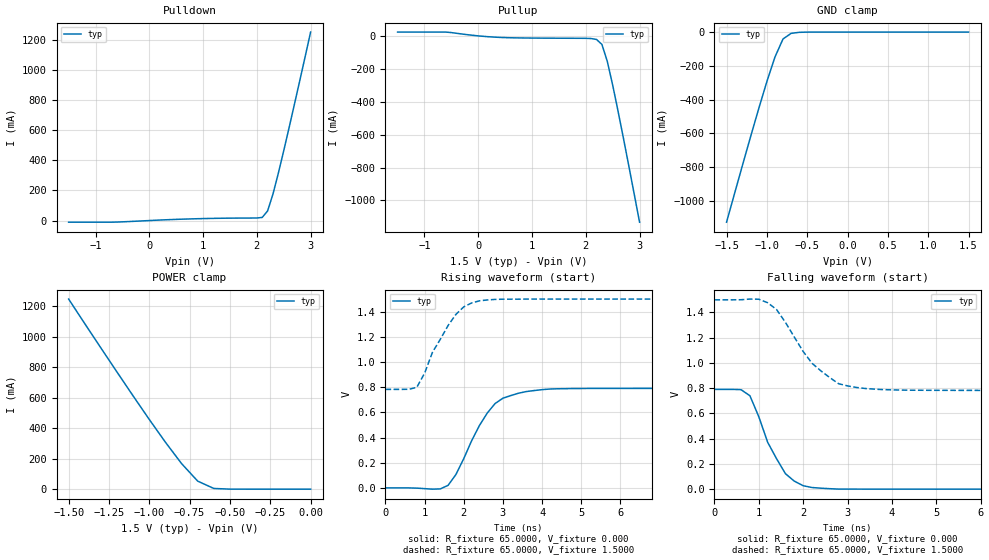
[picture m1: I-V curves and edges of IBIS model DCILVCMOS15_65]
| / 7\'7
| \ \   Xilinx Inc.
| / /
| \_\/.\   IBIS Model for Virtex-II
[IBIS ver]   2.1
[File name]   dci1565.ibs
[File Rev]   1.1
[Date]   Aug. 1, 2001
[Source]   Hspice simulations (08-01: TT, SS, FF)
[Notes]   Xilinx IBIS model for LVDCI 1.5V 65 ohms driver
[Disclaimer] The data in this model is derived from SPICE simulations using
   modeling information extracted from the target process. While
   a great deal of care has been taken to provide information
   that is accurate, this model is considered preliminary as it
   has not been verified by actual silicon measurement. Treat the
   data in this model as preliminary until actual silicon
   verification is performed.
[Copyright]   Copyright 2001, Xilinx Inc., All rights reserved
|   Component Virtex_II
[Component]   Virtex_II
[Manufacturer]   Xilinx Inc.
[Package]
| variable   typ   min   max
R_pkg   0.1000   NA   NA
L_pkg   0.8000nH   NA   NA
C_pkg   0.5000pF   NA   NA
[Pin]  signal_name   model_name   R_pin   L_pin   C_pin
io   DCILVCMOS15_65   DCILVCMOS15_65
| ins  insig   inp
| ens  ensig   inp
PGND   GND   GND
VCCO   VCCO   POWER
| Models and submodels in the file (1): DCILVCMOS15_65 (I/O)
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|   Model DCILVCMOS15_65
[Model]   DCILVCMOS15_65
Model_type   I/O
Polarity   Non-Inverting
Enable   Active-Low
Vinh = 1.05V
Vinl = 0.3V
Vmeas =   0.7300V
Cref =  35.0000pF
Rref =   1.0000M
Vref =  0.000V
C_comp   7.0000pF   NA   NA
[Temperature Range]   25.0000   NA   NA
[Voltage Range]   1.5000V   NA   NA
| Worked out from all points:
|   slope of the pulldown table from 0 to 0.225 V, typ, clamps not added: 58.8 ohm
|   slope of the pullup table from 0 to 0.225 V, typ, clamps not added: 37.5 ohm
|   GND clamp passes 1 mA (typ) near -0.57 V on its own axis
|   POWER clamp passes 1 mA (typ) near -0.52 V on its own axis
|   rising waveform, R_fixture 65.0000, V_fixture 0.000: 20-80 % time 819ps typ, NA min, NA max; typ from 0 V to 0.79 V
|   rising waveform, R_fixture 65.0000, V_fixture 1.5000: 20-80 % time 732ps typ, NA min, NA max; typ from 0.782 V to 1.5 V
|   falling waveform, R_fixture 65.0000, V_fixture 0.000: 20-80 % time 611ps typ, NA min, NA max; typ from 0.79 V to 0 V
|   falling waveform, R_fixture 65.0000, V_fixture 1.5000: 20-80 % time 911ps typ, NA min, NA max; typ from 1.5 V to 0.782 V
[Pulldown]
| voltage   I(typ)   I(min)   I(max)
-1.5V     -10.89mA   NA         NA
-700mV    -10.89mA   NA         NA
700mV     10.17mA    NA         NA
2.1V      20.64mA    NA         NA
2.2V      63.82mA    NA         NA
2.3V      175.9mA    NA         NA
2.4V      314.8mA    NA         NA
2.6V      617.3mA    NA         NA
3V        1.252A     NA         NA
[Pullup]
| voltage   I(typ)   I(min)   I(max)
-1.5V     22.99mA    NA         NA
-600mV    22.99mA    NA         NA
0V        -4.6nA     NA         NA
400mV     -9.254mA   NA         NA
2V        -14.9mA    NA         NA
2.2V      -21.92mA   NA         NA
2.3V      -52.01mA   NA         NA
2.4V      -155.2mA   NA         NA
2.5V      -299.2mA   NA         NA
2.6V      -457.5mA   NA         NA
2.8V      -790.2mA   NA         NA
3V        -1.132A    NA         NA
[GND_clamp]
| voltage   I(typ)   I(min)   I(max)
-1.5V     -1.127A    NA         NA
-1.2V     -617mA     NA         NA
-1V       -293.4mA   NA         NA
-900mV    -148mA     NA         NA
-800mV    -41mA      NA         NA
-700mV    -7.588mA   NA         NA
-600mV    -1.413mA   NA         NA
1.5V      218.4nA    NA         NA
[POWER_clamp]
| voltage   I(typ)   I(min)   I(max)
-1.5V     1.246A     NA         NA
-1.1V     610.9mA    NA         NA
-900mV    307.7mA    NA         NA
-800mV    167.8mA    NA         NA
-700mV    52.78mA    NA         NA
-600mV    4.607mA    NA         NA
0V        218.4nA    NA         NA
[Ramp]
| variable   typ   min   max
dV/dt_r   0.4743/0.8211n   NA   NA
dV/dt_f   0.4305/0.9045n   NA   NA
R_load = 65.0000
[Rising Waveform]
R_fixture = 65.0000
V_fixture = 0.000
| time   V(typ)   V(min)   V(max)
0s        10.73uV    NA         NA
1.4ns     -8.408mV   NA         NA
1.6ns     20.23mV    NA         NA
1.8ns     106.7mV    NA         NA
2.2ns     373.9mV    NA         NA
2.6ns     594.6mV    NA         NA
3ns       712.4mV    NA         NA
3.4ns     752.2mV    NA         NA
4.4ns     787.3mV    NA         NA
10ns      790.5mV    NA         NA
[Rising Waveform]
R_fixture = 65.0000
V_fixture = 1.5000
V_fixture_min = 1.4000
V_fixture_max = 1.6000
| time   V(typ)   V(min)   V(max)
0s        782.5mV    NA         NA
800ps     798.9mV    NA         NA
1ns       911.4mV    NA         NA
1.2ns     1.077V     NA         NA
1.6ns     1.29V      NA         NA
1.8ns     1.379V     NA         NA
2ns       1.438V     NA         NA
2.4ns     1.486V     NA         NA
3ns       1.499V     NA         NA
10ns      1.5V       NA         NA
[Falling Waveform]
R_fixture = 65.0000
V_fixture = 0.000
| time   V(typ)   V(min)   V(max)
0s        790.5mV    NA         NA
600ps     788.2mV    NA         NA
800ps     739.8mV    NA         NA
1ns       573.8mV    NA         NA
1.2ns     371.1mV    NA         NA
1.4ns     241.4mV    NA         NA
1.6ns     122.7mV    NA         NA
2ns       27.27mV    NA         NA
2.8ns     594.3uV    NA         NA
10ns      -6.526uV   NA         NA
[Falling Waveform]
R_fixture = 65.0000
V_fixture = 1.5000
V_fixture_min = 1.4000
V_fixture_max = 1.6000
| time   V(typ)   V(min)   V(max)
0s        1.5V       NA         NA
1ns       1.505V     NA         NA
1.2ns     1.477V     NA         NA
1.4ns     1.423V     NA         NA
2ns       1.091V     NA         NA
2.2ns     997.3mV    NA         NA
2.8ns     835.1mV    NA         NA
3ns       818.2mV    NA         NA
4.2ns     785mV      NA         NA
10ns      782.5mV    NA         NA
